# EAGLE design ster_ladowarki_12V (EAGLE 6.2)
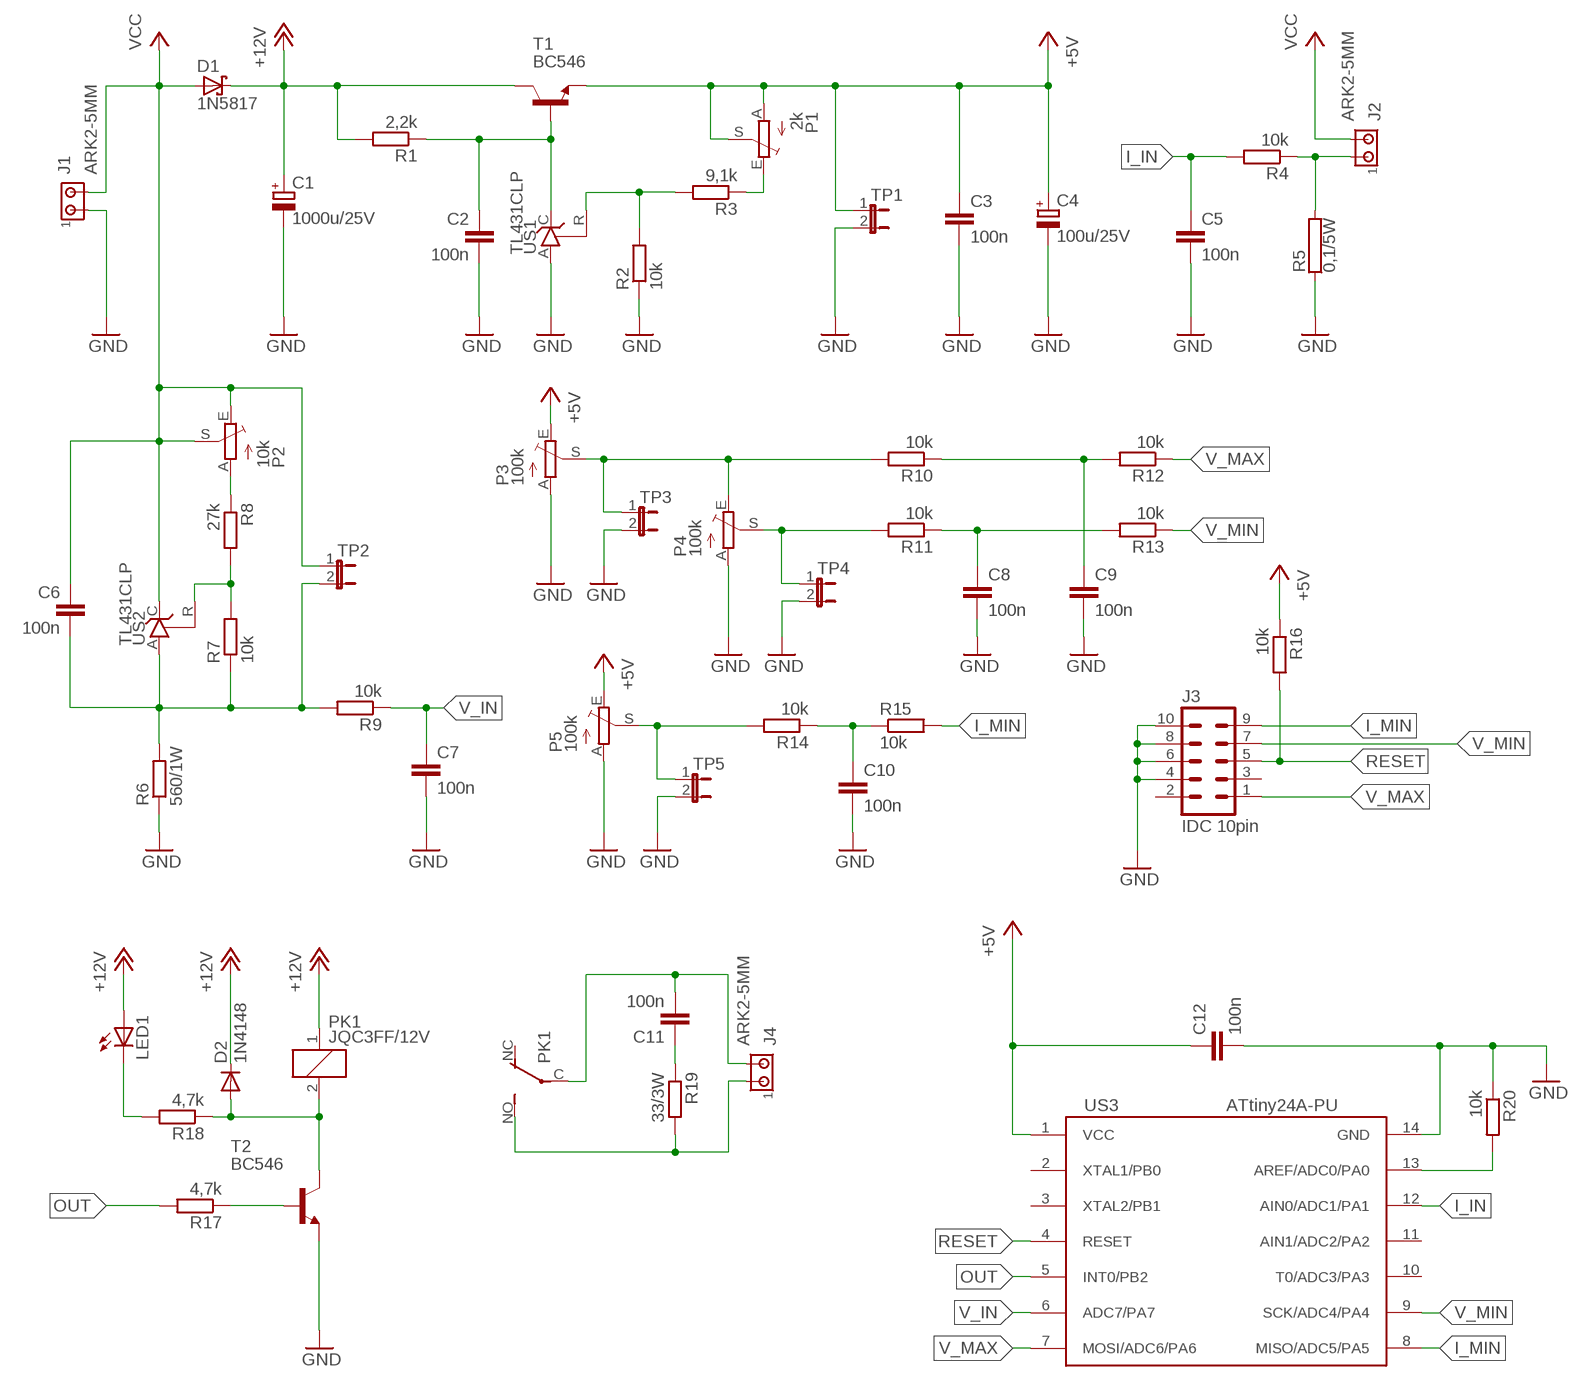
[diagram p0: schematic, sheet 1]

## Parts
C1  1000u/25V  CPOL-EUE5-10.5  [E5-10,5]
C2  100n  C-EU050-030X075  [C050-030X075]
C3  100n  C-EU050-030X075  [C050-030X075]
C4  100u/25V  CPOL-EUE2.5-6  [E2,5-6]
C5  100n  C-EU050-030X075  [C050-030X075]
C6  100n  C-EU050-030X075  [C050-030X075]
C7  100n  C-EU050-030X075  [C050-030X075]
C8  100n  C-EU050-030X075  [C050-030X075]
C9  100n  C-EU050-030X075  [C050-030X075]
C10  100n  C-EU050-030X075  [C050-030X075]
C11  100n  C-EU102_152-062X184  [C102_152-062X184]
C12  100n  C-EU050-030X075  [C050-030X075]
D1  1N5817  BAT49  [DO41-10]
D2  1N4148  1N4148DO35-7  [DO35-7]
J1  ARK2-5MM  [2PIN-5MM]
J2  ARK2-5MM  [2PIN-5MM]
J3  IDC 10pin  ML10  [ML10]
J4  ARK2-5MM  [2PIN-5MM]
LED1  LED5MM  [LED5MM]
P1  2k  TRIM_EU-PTSPIN  [PT-SPIN]
P2  10k  TRIM_EU-PTSPIN  [PT-SPIN]
P3  100k  TRIM_EU-PTSPIN  [PT-SPIN]
P4  100k  TRIM_EU-PTSPIN  [PT-SPIN]
P5  100k  TRIM_EU-PTSPIN  [PT-SPIN]
PK1  JQC3FF/12V  PK_POJED-JQC-3FG  [PK_POJED_JQC-3FG]
R1  2,2k  R-EU_0207/7  [0207/7]
R2  10k  R-EU_0207/7  [0207/7]
R3  9,1k  R-EU_0207/7  [0207/7]
R4  10k  R-EU_0207/7  [0207/7]
R5  0,1/5W  R-5W  [R_5W]
R6  560/1W  R-EU_0309/12  [0309/12]
R7  10k  R-EU_0207/7  [0207/7]
R8  27k  R-EU_0207/7  [0207/7]
R9  10k  R-EU_0207/7  [0207/7]
R10  10k  R-EU_0207/7  [0207/7]
R11  10k  R-EU_0207/7  [0207/7]
R12  10k  R-EU_0207/7  [0207/7]
R13  10k  R-EU_0207/7  [0207/7]
R14  10k  R-EU_0207/7  [0207/7]
R15  10k  R-EU_0207/7  [0207/7]
R16  10k  R-EU_0207/7  [0207/7]
R17  4,7k  R-EU_0207/7  [0207/7]
R18  4,7k  R-EU_0207/7  [0207/7]
R19  33/3W  R-EU_0617/5V  [0617V]
R20  10k  R-EU_0207/7  [0207/7]
T1  BC546  BC546A  [TO92-EBC]
T2  BC546  BC546A  [TO92-EBC]
TP1  JP1E  [JP1]
TP2  JP1E  [JP1]
TP3  JP1E  [JP1]
TP4  JP1E  [JP1]
TP5  JP1E  [JP1]
US1  TL431CLP  [TO92-CLP]
US2  TL431CLP  [TO92-CLP]
US3  ATtiny24A-PU  ATTINY24/44/84-PU  [DIL14]

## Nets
+5V: C3.1 C4.+ C12.1 P1.A P1.S P3.E P5.E R16.1 T1.E TP1.1 US3.1(VCC)
+12V: C1.+ D1.C D2.C LED1.A PK1.1 R1.2 T1.C
GND: C1.- C2.2 C3.2 C4.- C5.2 C7.2 C8.2 C9.2 C10.2 C12.2 J1.P$1 J3.4 J3.6 J3.8 J3.10 P3.A P4.A P5.A R2.1 R5.P$1 R6.1 R20.1 T2.E TP1.2 TP3.2 TP4.2 TP5.2 US1.A US3.14(GND)
I_IN: C5.1 R4.2 US3.12(AIN0/ADC1/PA1)
I_MIN: J3.9 R15.2 US3.8(MISO/ADC5/PA5)
N$1: C2.1 R1.1 T1.B US1.C
N$2: R17.1 T2.B
N$3: LED1.K(C) R18.2
N$4: C8.1 R11.1 R13.2
N$5: J2.P$1 R4.1 R5.P$2
N$6: R20.2 US3.13(AREF/ADC0/PA0)
N$7: C9.1 R10.1 R12.2
N$8: C10.1 R14.1 R15.1
N$33: R2.2 R3.2 US1.R
N$34: P1.E R3.1
N$35: P3.S P4.E R10.2 TP3.1
N$36: C6.2 R6.2 R7.1 R9.2 TP2.2 US2.A
N$37: P4.S R11.2 TP4.1
N$38: R7.2 R8.2 US2.R
N$39: P2.A R8.1
N$40: P5.S R14.2 TP5.1
N$41: C11.1 R19.1
N$42: J4.P$1 PK1.NO R19.2
N$43: C11.2 J4.P$2 PK1.C(COM)
N$44: D2.A PK1.2 R18.1 T2.C
OUT: R17.2 US3.5(INT0/PB2)
RESET: J3.5 R16.2 US3.4(RESET)
V_IN: C7.1 R9.1 US3.6(ADC7/PA7)
V_MAX: J3.1 R12.1 US3.7(MOSI/ADC6/PA6)
V_MIN: J3.7 R13.1 US3.9(SCK/ADC4/PA4)
VCC: C6.1 D1.A J1.P$2 J2.P$2 P2.E P2.S TP2.1 US2.C
Unconnected: J3.2 J3.3 PK1.NC US3.2(XTAL1/PB0) US3.3(XTAL2/PB1) US3.10(T0/ADC3/PA3) US3.11(AIN1/ADC2/PA2)

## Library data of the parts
C1 C4 = rcl:CPOL-EU: POLARIZED CAPACITOR, European symbol
C2 C3 C5-C10 C12 = rcl:C-EU: CAPACITOR, European symbol
C11 = resistor:C-EU: CAPACITOR, European symbol
D1 = diode:BAT49: DIODE
D2 = diode:1N4148: DIODE
J1 J2 J4 = zlacza_futrzak:ARK2: ARK 2
J3 = con-harting-ml:ML10: HARTING; OC_FARNELL: unknown; OC_NEWARK: unknown
LED1 = led:LED: LED
P1-P5 = pot:TRIM_EU-: POTENTIOMETER
PK1 = inne_futrzak:PK_POJED
R1-R4 R6-R18 R20 = rcl:R-EU_: RESISTOR, European symbol
R5 = inne_futrzak:R
R19 = resistor:R-EU_: RESISTOR, European symbol
T1 T2 = transistor-npn:BC546*: NPN Transistor
TP1-TP5 = jumper:JP1E: JUMPER
US1 US2 = v-reg:TL431CLP: VOLTAGE REGULATOR
US3 = scalaki_futrzak:ATTINY24/44/84

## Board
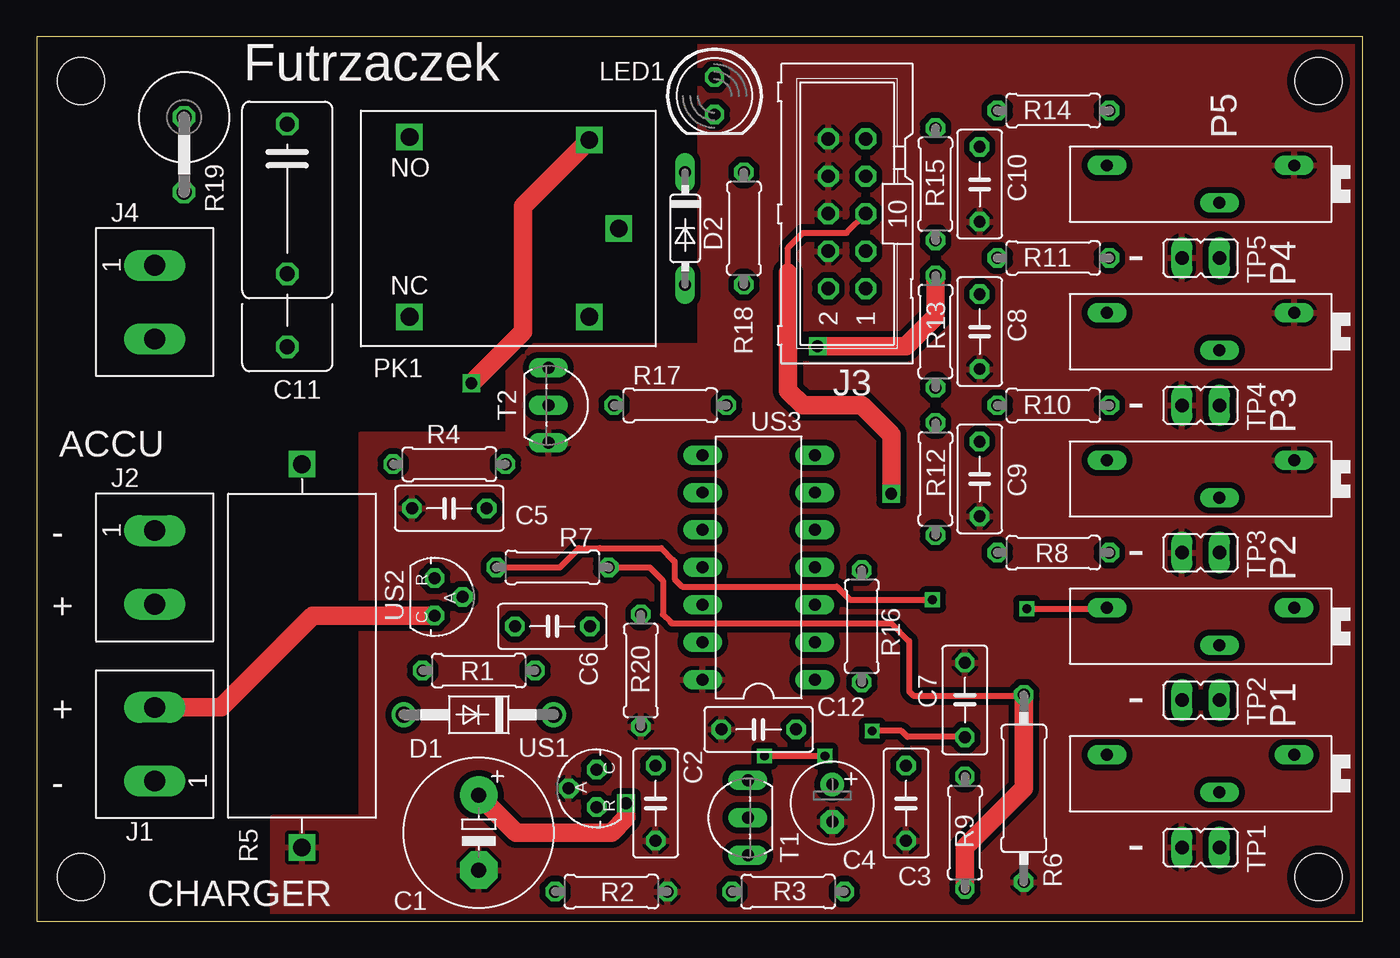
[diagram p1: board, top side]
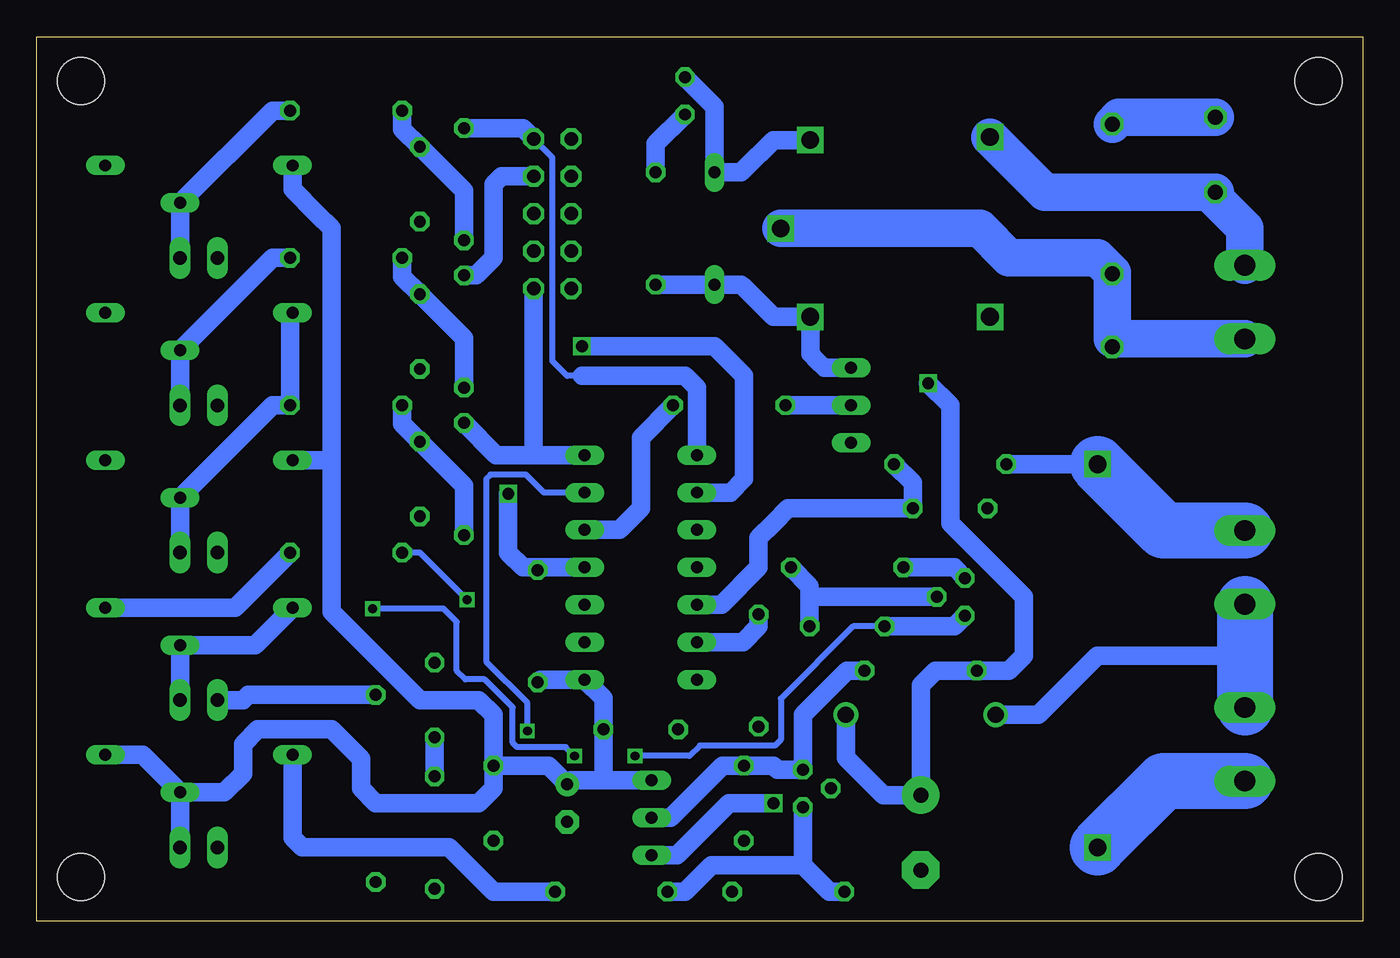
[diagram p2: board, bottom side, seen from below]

Size 90 x 60 mm. Coordinates in mm from the lower left corner, seen from the top.
Outline: 0,0 90,0 90,60 0,60 0,0
Copper layers (1*16): Top 0.035mm / dielectric 1.5mm / Bottom 0.035mm
Design rules: minimum track width 10mil, minimum drill 23mil, track to track 8mil, track to pad 8mil, pad to pad 8mil, via to via 8mil, smd to smd 8mil, copper to edge 20mil, drill to drill 8mil, minimum pad ring 10mil, minimum via ring 8mil, stop-mask expansion 4mil, vias tented up to drill 0mil, thermal gap 10mil
Holes 3.2 mm at 3,3 3,57 87,3 87,57

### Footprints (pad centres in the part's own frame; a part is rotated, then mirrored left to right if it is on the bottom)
E5-10,5 = drill 1.016 pad 2.54: + -2.54,0 | drill 1.016 pad 2.54 octagon: - 2.54,0
C050-030X075 = drill 0.813 octagon: 1 -2.54,0; 2 2.54,0
E2,5-6 = drill 0.813 pad 1.6: + -1.27,0 | drill 0.813 pad 1.6 octagon: - 1.27,0
C102_152-062X184 = drill 1.016 octagon: 1 -5.08,0; 2 5.08,0; 3 10.033,0
DO41-10 = drill 1.118: A 5.08,0; C -5.08,0
DO35-7 = drill 0.813 long: A 3.81,0; C -3.81,0
2PIN-5MM = drill 1.4 long: P$1 -2.5,0; P$2 2.5,0
ML10 = drill 0.914 octagon: 1 -5.08,-1.27; 2 -5.08,1.27; 3 -2.54,-1.27; 4 -2.54,1.27; 5 0,-1.27; 6 0,1.27; 7 2.54,-1.27; 8 2.54,1.27; 9 5.08,-1.27; 10 5.08,1.27
LED5MM = drill 0.813 octagon: A -1.27,0; K 1.27,0
PT-SPIN = drill 0.813 long: A -6.35,-1.27; E 6.35,-1.27; S -1.27,1.27
PK_POJED_JQC-3FG = drill 1.2 square: 1 5.5,6; 2 5.5,-6; C 7.5,0; NC -6.7,-6; NO -6.7,6.2
0207/7 = drill 0.813 octagon: 1 -3.81,0; 2 3.81,0
R_5W = drill 1.2 square: P$1 -13,0; P$2 13,0
0309/12 = drill 0.813 octagon: 1 -6.35,0; 2 6.35,0
0617V = drill 1.016 octagon: 1 -2.54,0; 2 2.54,0
TO92-EBC = drill 0.813 long: B 0,-1.27; C -2.54,-1.27; E 2.54,-1.27
JP1 = drill 0.914 long: 1 0,-1.27; 2 0,1.27
TO92-CLP = drill 0.813 octagon: A 0,1.905; C 1.27,0; R -1.27,0
DIL14 = drill 0.813 long: 1 -7.62,-3.81; 2 -5.08,-3.81; 3 -2.54,-3.81; 4 0,-3.81; 5 2.54,-3.81; 6 5.08,-3.81; 7 7.62,-3.81; 8 7.62,3.81; 9 5.08,3.81; 10 2.54,3.81; 11 0,3.81; 12 -2.54,3.81; 13 -5.08,3.81; 14 -7.62,3.81

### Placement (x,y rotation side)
C1  30,6 270 top
C2  42,8 270 top
C3  59,8 270 top
C4  54,8 270 top
C5  28,28 180 top
C6  35,20 0 top
C7  63,15 90 top
C8  64,40 270 top
C9  64,30 270 top
C10  64,50 270 top
C11  17,49 270 top
C12  49,13 180 top
D1  30,14 180 top
D2  44,47 270 top
J1  8,12 90 top
J2  8,24 270 top
J3  55,48 90 top
J4  8,42 270 top
LED1  46,56 270 top
P1  79,10 180 top
P2  79,20 180 top
P3  79,30 180 top
P4  79,40 180 top
P5  79,50 180 top
PK1  32,47 0 top
R1  30,17 180 top
R2  39,2 180 top
R3  51,2 180 top
R4  28,31 0 top
R5  18,18 90 top
R6  67,9 90 top
R7  35,24 180 top
R8  69,25 180 top
R9  63,6 270 top
R10  69,35 0 top
R11  69,45 0 top
R12  61,30 270 top
R13  61,40 270 top
R14  69,55 0 top
R15  61,50 90 top
R16  56,20 90 top
R17  43,35 0 top
R18  48,47 90 top
R19  10,52 270 top
R20  41,17 90 top
T1  47,7 90 top
T2  36,35 270 top
TP1  79,5 90 top
TP2  79,15 90 top
TP3  79,25 90 top
TP4  79,35 90 top
TP5  79,45 90 top
US1  38,9 90 top
US2  27,22 270 top
US3  49,24 90 top

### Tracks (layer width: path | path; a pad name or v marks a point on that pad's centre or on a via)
+5V
  Bottom 1.27: T1.E 51,9.54 | 51,9.54 53.73,9.54 C4.+ 55.27,10.54 C3.1 | 51,9.54 51.54,9.54 C12.1 51.54,15.11 US3.1 55.81,16.38 R16.1 | C3.1 59,9 60,8 67,8 68,9 68,11 70,13 75,13 76,12 76,10 77.27,8.73 P1.S | P1.A 82.81,11.27 P1.S | P1.S TP1.1 | P5.E 72.65,49.65 71,48 70,47 70,31 | 70,31 70,21 64,15 60,15 59,14 C3.1 | P3.E 70.27,31.27 70,31
+12V  (via drill 0.8)
  Top 1.27: PK1.1 33,48.5 33,40.5 33,40 v29.5,36.5 | v40,8 40,7 39,6 32.54,6 C1.+
  Bottom 1.27: D1.C 35.08,11.08 33,9 32.54,8.54 C1.+ 30,16 29,17 R1.2 24,17 23,18 23,22 28,27 28,34 28,35 v29.5,36.5 | PK1.1 40,53 42,51 42.19,50.81 D2.C 44,55.27 LED1.A | T1.C 46.54,4.46 43,8 42,8 v40,8
GND
  Bottom 3.81: J1.P$1 13.5,9.5 R5.P$1
  pour Top (isolate 0.406): 90,0 90,60 45,60 45,39 32,39 32,33 22,33 22,7 16,7 16,0
I_IN
  Bottom 1.27: R4.2 30.54,29.73 C5.1 39,28 40,27 41,26 41,24 43.54,21.46 US3.12
I_MIN
  Bottom 0.406: 53,37 54,37 55,38 55,51.81 J3.9
  Bottom 1.27: US3.8 45.19,36.19 46,37 53,37 | R15.2 57,53.81 J3.9
N$1
  Bottom 1.27: R1.1 35,17 38,14 US1.C 39.73,10.27 40,10.54 C2.1 43.46,10.54 47,7 T1.B
N$2
  Bottom 1.27: T2.B R17.1
N$3
  Bottom 1.27: R18.2 48,52.73 LED1.K
N$4
  Bottom 1.27: R11.1 65.19,43.73 C8.1 61,39.54 R13.2
N$5
  Bottom 1.27: R5.P$2 R4.1
  Bottom 3.81: J2.P$1 13.5,26.5 R5.P$2
N$6
  Bottom 1.27: US3.13 42.08,18.92 41,20 R20.2
N$7
  Bottom 1.27: R10.1 65.19,33.73 C9.1 61,29.54 R12.2
N$8
  Bottom 1.27: R14.1 65.19,53.73 C10.1 61,49.54 R15.1
N$33
  Bottom 1.27: US1.R 38,4.81 38,3.8 | R3.2 46,2 45,3 44.2,3.8 38.81,3.8 38,3.8 | R2.2 36.2,2 38,3.8
N$34
  Bottom 1.27: P1.E 72.65,5.65 72,5 62,5 59,2 R3.1
N$35
  Bottom 1.27: TP3.1 P3.S 74,35 R10.2 72.81,41.11 P4.E
N$36
  Top 0.406: R7.1 41.6,24 42.5,23.1 42.5,20.8 43,20.3 43.1,20.2 58,20.2 59.2,19 59.2,15.6 59.5,15.3 66.95,15.3 R6.2
  Top 1.27: R6.2 67,9 63,5 R9.2
  Bottom 1.27: C6.2 37.54,22 | 37.54,22 37.54,22.73 R7.1 | US2.A 37.54,22 | R6.2 75.65,15.35 76,15 TP2.2
N$37
  Bottom 1.27: R11.2 74,45 P4.S TP4.1
N$38  (via drill 0.6)
  Top 0.406: R7.2 35.5,24 36.8,25.3 38.2,25.3 42.4,25.3 43.2,24.5 43.3,24.4 43.3,23.2 43.8,22.7 54.3,22.7 55.2,21.8 v60.8,21.8
  Bottom 0.406: v60.8,21.8 64,25 R8.2
  Bottom 1.27: R7.2 27.73,24 US2.R
N$39
  Bottom 1.27: P2.A 76.54,21.27 R8.1
N$40
  Bottom 1.27: TP5.1 P5.S 74,55 R14.2
N$41
  Bottom 2.54: R19.1 16.54,54.54 C11.1
N$42
  Bottom 2.54: J4.P$1 8,47 10,49 R19.2 21.56,49.46 PK1.NO
N$43
  Bottom 2.54: J4.P$2 17,39.5 C11.2 17,44 18,45 24,45 26,47 PK1.C
N$44
  Bottom 1.27: R18.1 D2.A 42.19,43.19 42,43 40,41 PK1.2 37.5,38.5 37,38 36.54,37.54 T2.C
OUT
  Bottom 1.27: R17.2 49,32.81 49,30 49,28 50.46,26.54 US3.5
RESET  (via drill 0.8)
  Top 0.406: 51,44 51,45.7 52,46.7 54.97,46.7 J3.5
  Top 1.27: v58,29 58,33 56,35 52,35 51,36 51,44
  Bottom 1.27: US3.4 55.81,24 | 55.81,24 R16.2 | 55.81,24 57,24 58,25 v58,29
V_IN  (via drill 0.6)
  Top 0.406: C7.1 62.96,12.5 59.1,12.5 58.7,12.9 v56.7,12.9
  Bottom 0.406: US3.6 55.58,29.08 56.8,30.3 59.2,30.3 59.5,30 59.5,17.6 56.7,14.8 v56.7,12.9
  Bottom 1.27: R9.1 C7.1
V_MAX
  Bottom 1.27: US3.7 56,31.62 | 56,31.62 58.81,31.62 R12.1 | J3.1 56.27,31.62 56,31.62
V_MIN  (via drill 0.8)
  Top 1.27: v53,39 59,39 61,41 R13.1
  Bottom 1.27: US3.9 42.92,29.08 42,30 42,37 44,39 51,39 v53,39 | J3.7 58.46,50.54 59,50 59,45 60,44 60.19,43.81 R13.1
VCC  (via drill 0.6)
  Top 0.406: v49.4,11.2 v53.5,11.2 | v67.2,21.2 72.58,21.2 P2.E
  Top 1.27: US2.C 18.73,20.73 13,15 12.5,14.5 J1.P$2
  Bottom 0.406: C6.1 34.6,20 39.5,15.1 39.5,12.3 39.9,11.9 45,11.9 45.7,11.2 v49.4,11.2 | v53.5,11.2 54.1,11.8 57.4,11.8 57.7,12.1 57.7,14.5 59.6,16.4 60.9,16.4 61.5,17 61.5,20.3 62.4,21.2 v67.2,21.2
  Bottom 1.27: D1.A 22,14 18,18 8,18 | C6.1 31,20 30,20 27.73,20 US2.C | TP2.1 P2.S 75.19,18.73 P2.E
  Bottom 3.81: J2.P$2 8,18 J1.P$2

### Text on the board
tPlace: Futrzaczek | - | - | ACCU | - | - | + | + | - | - | - | CHARGER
